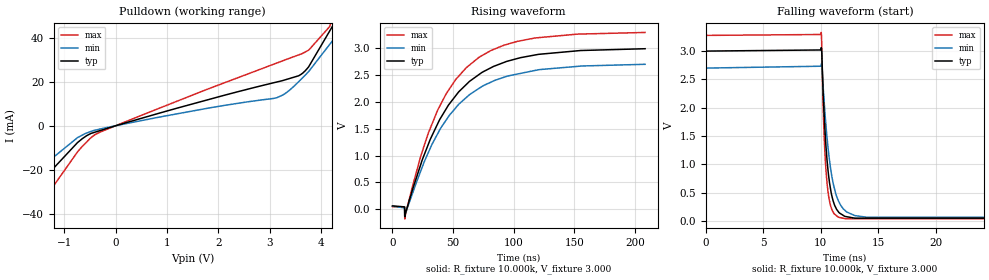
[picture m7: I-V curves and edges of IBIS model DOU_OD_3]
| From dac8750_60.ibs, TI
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|   DOU_OD Models
[Model] DOU_OD_3  |3V opem drain digital output
Model_type   Open_drain
Polarity   Non-Inverting
Vmeas = 1.5
Vref = 1.5
Cref = 0pF
Rref = 10000
|   typ   min   max
|   (nom PVT)   (Fast PVT)   (slow PVT)
|   ON state : BUFFER OUTPUT TURNED HIGH
C_comp   1.837E-12   1.691E-12   1.923E-12
|   OFF state: BUFFER OUTPUT TURNED LOW
|C_comp   1.746E-12   1.698E-12   1.862E-12
| Where   nom PVT is  Nominal Process, 3.0V, 36C
|   Fast PVT is Strong Process, 3.3V, -40C
|   Slow PVT is Weak Process, 2,7V, 134C
|C_comp - from L-C Tank method, L = 1nH, peak frequency
[Voltage Range]   3   2.7   3.3
|Operating Temperature   27   125   -40
|Junction Temperature
[Temperature Range]   36   134   -40
[Pullup Reference]   3   2.7   3.3
[Pulldown Reference]   0   0   0
[Power Clamp Reference]   3   2.7   3.3
[GND Clamp Reference]   0   0   0
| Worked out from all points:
|   slope of the pulldown table from 0 to 0.45 V, typ, clamps not added: 149 ohm
|   falling waveform, R_fixture 10.000k, V_fixture 3.000: 20-80 % time 612ps typ, 900ps min, 405ps max; typ from 3 V to 0.043 V
|   rising waveform, R_fixture 10.000k, V_fixture 3.000: 20-80 % time 44.3ns typ, 44.8ns min, 41.5ns max; typ from 0.061 V to 2.99 V
[Pulldown]
|   Voltage   I(typ)   I(min)   I(max)
-3V       -143.1mA   -86.11mA   -247.4mA
-2.367V   -72.85mA   -57.76mA   -92.85mA
-1.537V   -29.93mA   -20.56mA   -42.59mA
-1.379V   -23.6mA    -17.56mA   -33.02mA
-739.8mV  -7.642mA   -5.396mA   -11.87mA
-404.2mV  -2.946mA   -2.051mA   -4.106mA
3.138V    19.88mA    12.78mA    28.51mA
3.684V    24.92mA    22.94mA    33.47mA
4.157V    42.83mA    36.78mA    44.91mA
4.36V     50.91mA    42.9mA     56.16mA
4.581V    59.69mA    54.06mA    68.38mA
5.991V    154.6mA    125.2mA    189.8mA
[Ramp]
R_load = 10000
|   typ   min   max
dV/dt_r   1.75724/4.42651e-008   1.56122/4.45982e-008   1.94657/4.15617e-008
dV/dt_f   1.75631/6.08238e-010   1.56072/8.98126e-010   1.94568/4.0625e-010
[Falling Waveform]
R_fixture = 10.000k
V_fixture = 3.000
V_fixture_min = 2.700
V_fixture_max = 3.300
C_fixture = 0.000
|  time   V(typ)   V(min)   V(max)
0s        3V         2.7V       3.277V
10.04ns   3.05V      2.758V     3.329V
10.08ns   2.989V     2.759V     3.093V
10.19ns   2.334V     2.409V     2.101V
10.31ns   1.791V     2.046V     1.399V
10.45ns   1.305V     1.675V     884.4mV
10.64ns   868.7mV    1.274V     495.6mV
11.29ns   242.4mV    492.7mV    107.2mV
12.14ns   79.93mV    180.6mV    40.4mV
208.3ns   43.41mV    56.02mV    34.55mV
[Rising Waveform]
R_fixture = 10.000k
V_fixture = 3.000
V_fixture_min = 2.700
V_fixture_max = 3.300
C_fixture = 0.000
|  time   V(typ)   V(min)   V(max)
0s        61.42mV    56.02mV    48.82mV
10ns      43.39mV    24.14mV    34.55mV
10.14ns   -138.4mV   -120.5mV   -183.6mV
23.79ns   866.2mV    740.4mV    1.022V
36.84ns   1.572V     1.389V     1.824V
52.06ns   2.112V     1.886V     2.413V
71.09ns   2.505V     2.247V     2.825V
92ns      2.735V     2.459V     3.056V
117ns     2.871V     2.583V     3.188V
208.3ns   2.99V      2.7V       3.293V
